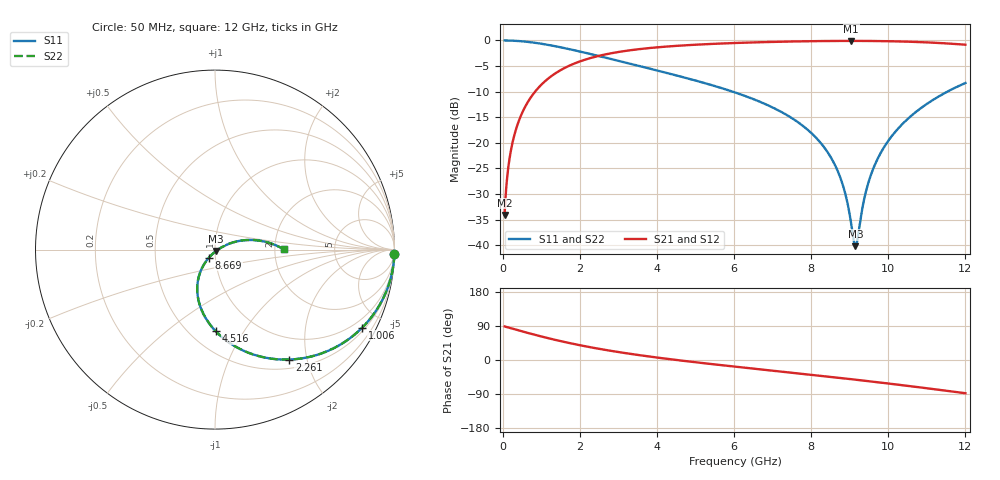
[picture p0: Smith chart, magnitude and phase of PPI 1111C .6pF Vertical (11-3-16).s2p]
# GHz S MA R 50
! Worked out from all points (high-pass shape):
!   1601 points, 50 MHz to 12 GHz, reference 50 ohm
!   highest |S21| = -0.09 dB at 9.035 GHz (marker M1); lowest = -34.1 dB at 50 MHz (marker M2)
!   |S21| within 3 dB of the highest: 2.451 GHz to end of sweep
!   lowest |S11| = -40.2 dB at 9.147 GHz (marker M3), VSWR 1.02, Z = 50.6 - j0.812 ohm
!   |S11| at or under -10 dB: 5.965 GHz to 11.53 GHz (5.567 GHz wide, 63.6 % of centre)
!   |S22| runs from -40.2 to 0.0 dB; largest |S21 - S12| = 0
!   S11 on the Smith chart (normalised r, x): 50 MHz: 1, -79; 1.006 GHz: 0.62, -3.93; 2.261 GHz: 0.63, -1.71; 4.516 GHz: 0.66, -0.76; 8.669 GHz: 0.93, -0.08; 12 GHz: 2.25, +0.01
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0.05  0.9998 -1.4  0.01982 88.6  0.01982 88.6  0.9998 -1.4
0.1844375  0.9973 -5.3  0.07293 84.7  0.07293 84.7  0.9973 -5.3
0.34875  0.9905 -10.0  0.137 80.0  0.137 80.0  0.9905 -10.0
0.6250938  0.9705 -17.8  0.2407 72.2  0.2407 72.2  0.9705 -17.8
1.006  0.9283 -27.9  0.3709 62.0  0.3709 62.0  0.9283 -27.9
2.044156  0.7731 -51.7  0.6322 38.1  0.6322 38.1  0.7731 -51.7
2.26075  0.7396 -55.9  0.6706 33.9  0.6706 33.9  0.7396 -55.9
4.038312  0.5054 -83.5  0.8587 6.0  0.8587 6.0  0.5054 -83.5
4.516312  0.4544 -89.5  0.8861 -0.1  0.8861 -0.1  0.4544 -89.5
6.025  0.3108 -106.4  0.9443 -17.5  0.9443 -17.5  0.3108 -106.4
7.205063  0.2025 -118.3  0.9717 -30.3  0.9717 -30.3  0.2025 -118.3
8.019156  0.1232 -125.4  0.9838 -39.2  0.9838 -39.2  0.1232 -125.4
8.668938  0.05524 -126.9  0.989 -46.4  0.989 -46.4  0.05524 -126.9
8.878063  0.03266 -122.1  0.9897 -48.8  0.9897 -48.8  0.03266 -122.1
9.034906  0.01655 -105.0  0.9898 -50.6  0.9898 -50.6  0.01655 -105.0
9.146937  0.00981 -54.9  0.9897 -51.9  0.9897 -51.9  0.00981 -54.9
9.199219  0.01134 -23.0  0.9896 -52.5  0.9896 -52.5  0.01134 -23.0
9.363531  0.02699 13.6  0.9891 -54.4  0.9891 -54.4  0.02699 13.6
9.520375  0.04516 20.5  0.9882 -56.3  0.9882 -56.3  0.04516 20.5
10.01331  0.1064 21.8  0.9827 -62.2  0.9827 -62.2  0.1064 21.8
10.83488  0.2168 14.3  0.9633 -72.4  0.9633 -72.4  0.2168 14.3
12  0.3842 0.2  0.9084 -87.7  0.9084 -87.7  0.3842 0.2
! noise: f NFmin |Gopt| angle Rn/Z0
0.05  0.001441  0.9804  1.367  0.01677
1.372  0.005855  0.7884  11.55  0.00564
2.701  0.009587  0.7466  18.75  0.00741
4.031  0.01303  0.728  26.04  0.009057
5.36  0.01639  0.7208  33.18  0.01071
6.682  0.01981  0.7212  40.02  0.01247
8.012  0.02342  0.7273  46.58  0.01448
9.341  0.02733  0.7381  52.81  0.01684
10.67  0.03167  0.7524  58.69  0.01973
12  0.03661  0.7695  64.25  0.02337
